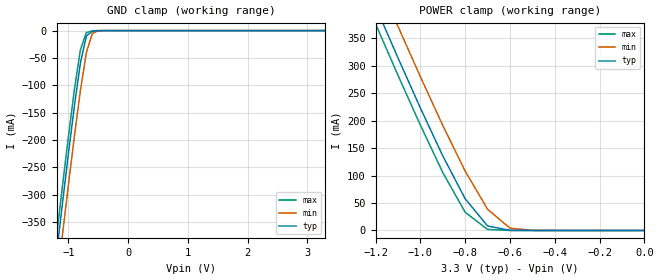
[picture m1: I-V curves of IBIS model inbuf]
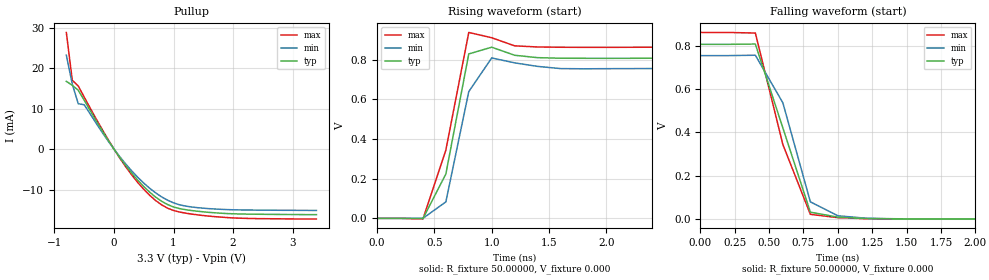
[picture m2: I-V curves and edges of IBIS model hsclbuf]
| IBIS file idt5v41066.ibs created by s2ibis2 version 1.2
| North Carolina State University Electronics Research Laboratory  1995
[IBIS ver]   2.1
[File name]   5v41066.ibs
[File Rev]   1.1
[Date]   May 3, 2012 Corrected non-monotonic warnings. lfp
|[File Rev]   1.0
|[Date]   July 19,2010
[Source]   IDT
[Notes]   1. Temp typ=25C, min=70C, max=0C 2. Ramp rates based on 50 ohm
   load
[Disclaimer] READ THESE TERMS AND CONDITIONS CAREFULLY BEFORE USING THIS
   IBIS MODEL. BY USING THIS IBIS MODEL, YOU ARE ACCEPTING AND
   AGREEING TO THESE TERMS AND CONDITIONS OF USE. Integrated
   Device Technology, Inc. ("IDT") hereby grants the user of this
   IBIS model ("User") a non-exclusive, nontransferable license
   to use this IBIS model under the following terms: The User is
   granted this license only to use the IBIS model for
   demonstration purposes only and is not granted rights to sell,
   copy (except as needed to run the IBIS model), rent, lease or
   sub-license (except for demonstration) the IBIS model in whole
   or in part, or in modified form to anyone. The User may modify
   the IBIS model to suit its specific applications, but rights
   to derivative works and such modifications shall belong to
   IDT. THIS IBIS MODEL IS PROVIDED ON AN AS IS" BASIS AND IDT
   MAKES ABSOLUTELY NO WARRANTY WITH RESPECT TO THE INFORMATION
   CONTAINED HEREIN. IDT DISCLAIMS AND USER WAIVES ALL
   WARRANTIES, EXPRESS AND IMPLIED, INCLUDING WARRANTIES OF
   MERCHANTABILITY AND FITNESS FOR A PARTICULAR PURPOSE. THE
   ENTIRE RISK AS TO QUALITY AND PERFORMANCE IS WITH THE USER
   ACCORDINGLY, IN NO EVENT SHALL IDT BE LIABLE FOR ANY DIRECT OR
   INDIRECT DAMAGES, WHETHER IN CONTRACT OR TORT, INCLUDING ANY
   LOST PROFITS OR OTHER INCIDENTAL, CONSEQUENTIAL, EXEMPLARY, OR
   PUNITIVE DAMAGES ARISING OUT OF THE USE OR APPLICATION OF THE
   IBIS MODEL, WHETHER OR NOT IDT HAD NOTICE OF SUCH DAMAGES. IDT
   reserves the right to make changes without notice to any
   product herein to improve reliability, function, or design.
   IDT does not convey any license under patent rights or any
   other intellectual property rights, including those of third
   parties. IDT is not obligated to provide maintenance or
   support for the licensed IBIS model.
   ******* This model is for the IDT5V41066*********************
[Copyright]   Copyright 2010, Integrated Device Technology, Inc. All rights
   reserved.
|   Component IDT5V41066
[Component]   IDT5V41066
[Manufacturer]   Integrated Device Technology Inc.
[Package]
| variable   typ   min   max
R_pkg   81.10000m   62.20000m   100.00000m
L_pkg   6.70000nH   4.90000nH   8.50000nH
C_pkg   0.53000pF   0.21000pF   0.85000pF
[Pin]  signal_name   model_name   R_pin   L_pin   C_pin
1   VDDXD   POWER
2   S0   inbuf
3   S1   inbuf
4   S2   inbuf
5   X1   NC
6   X2   NC
7   PDB   inbuf
8   OE   inbuf
9   GNDXD   GND
10   IREF   NC
11   CLKDB   hsclbuf
12   CLKD   hsclbuf
13   CLKCB   hsclbuf
14   CLKC   hsclbuf
15   VDDODA   POWER
16   GNDODA   GND
17   CLKBB   hsclbuf
18   CLKB   hsclbuf
19   CLKAB   hsclbuf
20   CLKA   hsclbuf
| in   in   dummy
| oe   oe   dummy
[Diff Pin]  inv_pin  vdiff   tdelay_typ  tdelay_min  tdelay_max
20   19   0.000V   0.000s   0.000s   0.000s
18   17   0.000V   0.000s   0.000s   0.000s
14   13   0.000V   0.000s   0.000s   0.000s
12   11   0.000V   0.000s   0.000s   0.000s
| Models and submodels in the file (2): inbuf (Input), hsclbuf (Open_source)
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|   Model inbuf
[Model]   inbuf
Model_type   Input
Vinl =  0.80000V
Vinh =  2.80000V
C_comp   3.40000pF   2.85000pF   3.95000pF
[Temperature Range]   25.00000   70.00000   0.000
[Voltage Range]   3.30000V   3.13500V   3.46500V
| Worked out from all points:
|   GND clamp passes 1 mA (typ) near -0.60 V on its own axis
|   POWER clamp passes 1 mA (typ) near -0.61 V on its own axis
[GND_clamp]
| voltage   I(typ)   I(min)   I(max)
-3.3V     -2.462A    -2.516A    -2.432A
-1.2V     -408.6mA   -466.1mA   -376.9mA
-1.1V     -315.3mA   -372.7mA   -283.7mA
-1V       -224.2mA   -281.2mA   -193mA
-900mV    -137.1mA   -192.5mA   -107.2mA
-800mV    -59.32mA   -109.4mA   -35.08mA
-700mV    -9.869mA   -39.95mA   -3.587mA
-600mV    -842uA     -5.099mA   -483.1uA
-500mV    -115.1uA   -371.4uA   -82.28uA
3.3V      126.6pA    4.065uA    -5.151uA
[POWER_clamp]
| voltage   I(typ)   I(min)   I(max)
-3.3V     2.461A     2.514A     2.431A
-1.2V     407.3mA    464.7mA    375.7mA
-1.1V     314mA      371.3mA    282.3mA
-1V       222.7mA    279.7mA    191.6mA
-900mV    135.6mA    191mA      105.4mA
-800mV    57.64mA    107.9mA    33.04mA
-700mV    8.171mA    38.53mA    1.847mA
-600mV    258.3uA    4.245mA    53.65uA
-500mV    21.3uA     185.2uA    18uA
0V        126.6pA    323.6pA    125.6pA
|   Model hsclbuf
[Model]   hsclbuf
Model_type   Open_source
Polarity   Non-Inverting
Enable   Active-High
Vmeas =  0.35000V
Rref = 50.00000
Vref =  0.000V
C_comp   3.40000pF   2.85000pF   3.95000pF
[Temperature Range]   25.00000   70.00000   0.000
[Voltage Range]   3.30000V   3.13500V   3.46500V
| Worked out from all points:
|   slope of the pullup table from 0 to 0.495 V, typ, clamps not added: 53.9 ohm
|   rising waveform, R_fixture 50.00000, V_fixture 0.000: 20-80 % time 195ps typ, 163ps min, 215ps max; typ from 0 V to 0.806 V
|   falling waveform, R_fixture 50.00000, V_fixture 0.000: 20-80 % time 249ps typ, 230ps min, 241ps max; typ from 0.806 V to 0 V
[Pullup]
| voltage   I(typ)   I(min)   I(max)
-800mV    16.74mA    23.22mA    28.82mA
-700mV    15.77mA    16.05mA    17mA
-600mV    14.54mA    11.21mA    15.6mA
-500mV    12.09mA    10.96mA    12.86mA
-200mV    4.592mA    4.177mA    4.901mA
100mV     -2.128mA   -1.929mA   -2.281mA
400mV     -7.7mA     -6.984mA   -8.261mA
700mV     -11.88mA   -10.83mA   -12.72mA
1V        -14.31mA   -13.29mA   -15.18mA
1.4V      -15.36mA   -14.48mA   -16.25mA
2.1V      -16.04mA   -15.04mA   -17.08mA
3.4V      -16.21mA   -15.18mA   -17.3mA
[Ramp]
| variable   typ   min   max
dV/dt_r   0.48390/0.14004n   0.45264/0.13312n   0.51678/0.11874n
dV/dt_f   0.48366/0.16100n   0.45247/0.17807n   0.51654/0.15404n
R_load = 50.00000
[Rising Waveform]
R_fixture = 50.00000
V_fixture = 0.000
V_fixture_min = 0.000
V_fixture_max = 0.000
| time   V(typ)   V(min)   V(max)
0s        0V         0V         0V
400ps     -1.245mV   110.3uV    -3.578mV
600ps     223.5mV    82.97mV    344.2mV
800ps     829mV      639.1mV    937.2mV
1ns       862.9mV    808.7mV    910.6mV
1.2ns     822.2mV    784mV      869.7mV
1.4ns     810.2mV    766.1mV    864mV
1.6ns     807.3mV    755mV      862.7mV
10ns      806.5mV    754.4mV    861.3mV
[Falling Waveform]
R_fixture = 50.00000
V_fixture = 0.000
V_fixture_min = 0.000
V_fixture_max = 0.000
| time   V(typ)   V(min)   V(max)
0s        806.1mV    754.1mV    860.9mV
400ps     807.4mV    755.9mV    858.2mV
600ps     420.4mV    536.3mV    343.8mV
800ps     31.73mV    79.3mV     21.64mV
1ns       8.713mV    15.08mV    6.327mV
1.2ns     2.276mV    3.998mV    1.628mV
1.4ns     807.5uV    1.469mV    357.8uV
10ns      -5.905uV   -12.28uV   6.645uV
